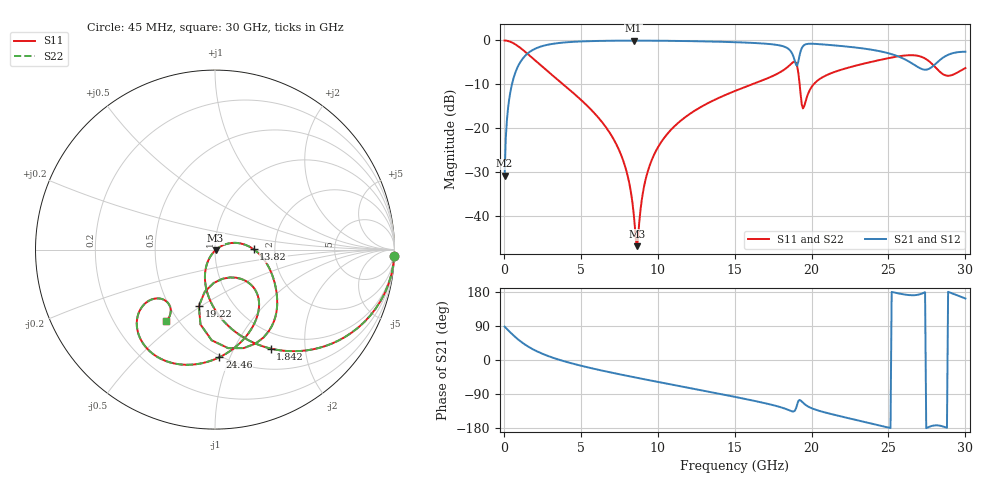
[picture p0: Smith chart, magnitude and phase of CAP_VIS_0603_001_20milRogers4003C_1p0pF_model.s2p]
! S-parameter model data by Modelithics Inc.  support@modelithics.com  813-866-6335  Tampa FL USA
! S-Parameter data specifications:
! Substrate: 20-mil Rogers 4003C, substrate thickness, H=0.508mm, Dielectric constant, Er=3.75
! PCB Mounting Pad Footprint: Pad width, PadW=0.90mm , Pad length, PadL=1.00mm , Pad gap, PadG (edge-to-edge)=1.00mm , Reference planes=3.0mm apart
! Created Wed Nov 18 13:17:32 2015
# hz S ma R 50
! 2 Port Network Data from SP1.SP block
! freq  magS11  angS11  magS21  angS21  magS12  angS12  magS22  angS22
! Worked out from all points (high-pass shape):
!   401 points, 45 MHz to 30 GHz, reference 50 ohm
!   highest |S21| = -0.05 dB at 8.432 GHz (marker M1); lowest = -30.9 dB at 45 MHz (marker M2)
!   |S21| within 3 dB of the highest: 1.519 GHz to 18.74 GHz (17.22 GHz wide, 170 % of centre); 19.25 GHz to 25.12 GHz (5.878 GHz wide, 26.5 % of centre)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
!   lowest |S11| = -46.9 dB at 8.657 GHz (marker M3), VSWR 1.01, Z = 50.4 - j0.286 ohm
!   |S11| at or under -10 dB: 3.848 GHz to 16.14 GHz (12.29 GHz wide, 123 % of centre); 19.22 GHz to 20.14 GHz (911.3 MHz wide, 4.63 % of centre)
!   |S22| runs from -46.9 to 0.0 dB; largest |S21 - S12| = 0
!   S11 on the Smith chart (normalised r, x): 45 MHz: 1, -61; 1.842 GHz: 0.77, -1.41; 13.82 GHz: 1.55, +0.01; 19.22 GHz: 0.69, -0.49; 24.46 GHz: 0.49, -0.91; 30 GHz: 0.43, -0.45
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4.5e7  0.9996 -1.9  0.02864 88.1  0.02864 88.1  0.9996 -1.9
2.696625e8  0.9855 -11.2  0.1694 78.8  0.1694 78.8  0.9855 -11.2
5.692125e8  0.9396 -23.1  0.3418 66.9  0.3418 66.9  0.9396 -23.1
1.8423e9  0.6323 -60.7  0.773 29.2  0.773 29.2  0.6323 -60.7
5.062462e9  0.206 -104.7  0.9749 -15.6  0.9749 -15.6  0.206 -104.7
7.458862e9  0.05761 -123.2  0.9936 -37.2  0.9936 -37.2  0.05761 -123.2
8.4324e9  0.01073 -111.1  0.9948 -45.2  0.9948 -45.2  0.01073 -111.1
8.657062e9  0.004508 -39.1  0.9948 -47.1  0.9948 -47.1  0.004508 -39.1
9.256162e9  0.02797 28.5  0.9941 -51.9  0.9941 -51.9  0.02797 28.5
1.007992e10  0.06328 27.1  0.9922 -58.4  0.9922 -58.4  0.06328 27.1
1.38243e10  0.2154 0.5  0.9686 -87.7  0.9686 -87.7  0.2154 0.5
1.50225e10  0.2654 -9.0  0.9552 -97.3  0.9552 -97.3  0.2654 -9.0
1.839244e10  0.4892 -45.7  0.824 -130.1  0.824 -130.1  0.4892 -45.7
1.891665e10  0.5716 -73.8  0.5799 -133.6  0.5799 -133.6  0.5716 -73.8
1.92162e10  0.3276 -106.0  0.6706 -105.5  0.6706 -105.5  0.3276 -106.0
1.951575e10  0.1762 -61.7  0.8839 -115.5  0.8839 -115.5  0.1762 -61.7
2.003996e10  0.3012 -44.5  0.917 -127.8  0.917 -127.8  0.3012 -44.5
2.445832e10  0.6 -87.6  0.7521 -173.2  0.7521 -173.2  0.6 -87.6
2.505742e10  0.6309 -94.9  0.7097 -179.0  0.7097 -179.0  0.6309 -94.9
2.737894e10  0.6223 -134.0  0.4637 178.8  0.4637 178.8  0.6223 -134.0
2.842736e10  0.4262 -140.3  0.6142 -174.1  0.6142 -174.1  0.4262 -140.3
3e10  0.4844 -124.3  0.7435 162.3  0.7435 162.3  0.4844 -124.3
